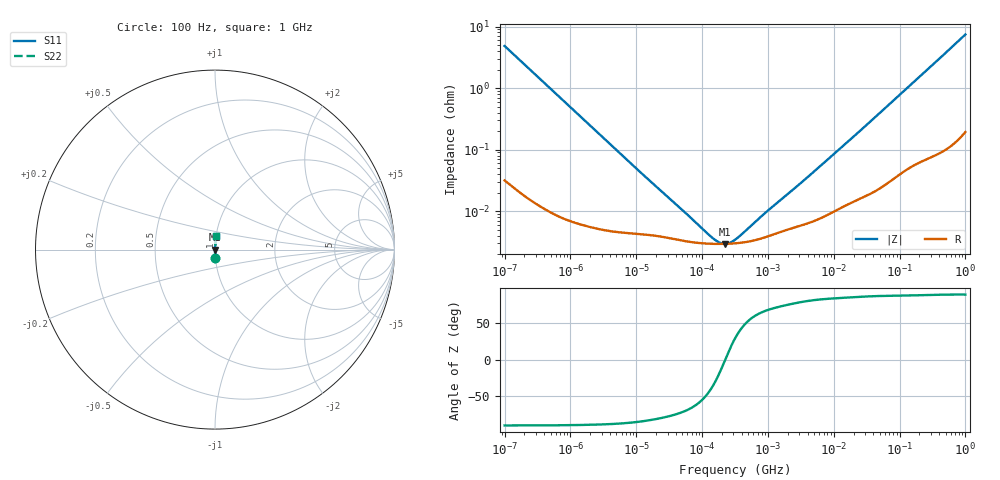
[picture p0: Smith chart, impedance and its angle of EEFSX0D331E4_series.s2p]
!  *** S-Parameter ***
!  Copyright (C) Panasonic Industry Corporation
!  Conductive Polymer Aluminum Electrolytic Capacitor (SP-Cap)
!  Parts No. EEFSX0D331E4
!  Connection Mode : Series
!  1  o---||---o  2
!  GND o--------o GND
!  Conditions : Temperature = 20 degC  DC Bias = 0 V
! Frequency Range : 100Hz  -  1GHz  [ 401 Steps ]
# Hz S RI R 50
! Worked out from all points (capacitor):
!   401 points, 100 Hz to 1 GHz, reference 50 ohm
!   read as one part in series: C = 329 uF near 108.4 Hz
!   lowest |Z| = 2.95 mohm at 220 kHz (marker M1)
!   series resonance near 224.8 kHz, so ESL is about 1.5 nH
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100  0.00264 -0.0481  0.9974 0.0481  0.9974 0.0481  0.00264 -0.0481
108.3927  0.00227 -0.0444  0.9977 0.0444  0.9977 0.0444  0.00227 -0.0444
296.8247  0.000399 -0.0163  0.9996 0.0163  0.9996 0.0163  0.000399 -0.0163
1487.647  7.08e-05 -0.00328  0.9999 0.00328  0.9999 0.00328  7.08e-05 -0.00328
8759.917  4.38e-05 -0.000562  1 0.000562  1 0.000562  4.38e-05 -0.000562
22130.95  3.92e-05 -0.000226  1 0.000226  1 0.000226  3.92e-05 -0.000226
47588.28  3.36e-05 -0.000105  1 0.000105  1 0.000105  3.36e-05 -0.000105
53703.18  3.28e-05 -9.23e-05  1 9.23e-05  1 9.23e-05  3.28e-05 -9.23e-05
58210.32  3.24e-05 -8.45e-05  1 8.45e-05  1 8.45e-05  3.24e-05 -8.45e-05
220039.2  2.95e-05 -1.02e-06  1 1.02e-06  1 1.02e-06  2.95e-05 -1.02e-06
316227.8  3.01e-05 1.65e-05  1 -1.65e-05  1 -1.65e-05  3.01e-05 1.65e-05
901571.1  3.76e-05 8.51e-05  1 -8.51e-05  1 -8.51e-05  3.76e-05 8.51e-05
977237.2  3.87e-05 9.25e-05  1 -9.25e-05  1 -9.25e-05  3.87e-05 9.25e-05
1059254  3.99e-05 0.0001  1 -0.0001  1 -0.0001  3.99e-05 0.0001
2676086  5.54e-05 0.00024  0.9999 -0.00024  0.9999 -0.00024  5.54e-05 0.00024
4704354  6.75e-05 0.000409  0.9999 -0.000409  0.9999 -0.000409  6.75e-05 0.000409
2.175204e7  0.000151 0.00176  0.9998 -0.00176  0.9998 -0.00176  0.000151 0.00176
6.99842e7  0.000328 0.00545  0.9997 -0.00545  0.9997 -0.00545  0.000328 0.00545
3.368992e8  0.00142 0.0251  0.9986 -0.0251  0.9986 -0.0251  0.00142 0.0251
5.688529e8  0.00287 0.0421  0.9971 -0.0421  0.9971 -0.0421  0.00287 0.0421
9.225714e8  0.00639 0.0679  0.9936 -0.0679  0.9936 -0.0679  0.00639 0.0679
1e9  0.00738 0.0735  0.9926 -0.0735  0.9926 -0.0735  0.00738 0.0735
